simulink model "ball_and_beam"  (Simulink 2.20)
settings: Solver=FixedStepDiscrete  StartTime=0.0  StopTime=5.0  FixedStep=0.02  RelTol=1e-3  AbsTol=1e-6

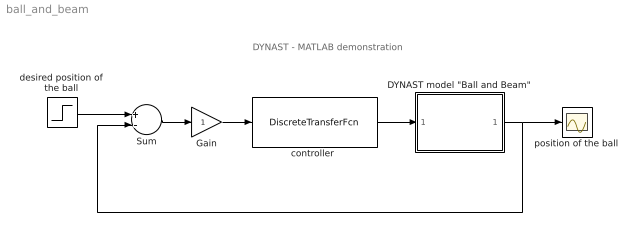
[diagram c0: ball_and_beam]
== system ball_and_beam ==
  note: DYNAST - MATLAB demonstration
  "DYNAST model \"Ball and Beam\"" : Subsystem
  Gain : Gain  Gain=1
  Sum : Sum  Inputs=+-
  "controller " : DiscreteTransferFcn  Numerator="[1010       -1020          10]"  Denominator="[1     1     0]"  SampleTime=0.02
  desired position of the ball : Step  Time=0  Before=0  After=0.25
  position of the ball : Scope
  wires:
  Sum/1 -> Gain/1
  Gain/1 -> "controller "/1
  "DYNAST model \"Ball and Beam\""/1(r) -> Sum/2, position of the ball/1
  "controller "/1 -> "DYNAST model \"Ball and Beam\""/1(theta)
  desired position of the ball/1 -> Sum/1

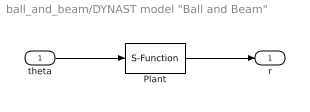
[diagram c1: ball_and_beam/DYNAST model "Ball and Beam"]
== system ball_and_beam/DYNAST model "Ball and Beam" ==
  theta : Inport  Port=1  PortWidth=-1  SampleTime=-1
  Plant : S-Function  FunctionName=dynPlantL  Parameters='%DYNAST%\examples\control\BallBeam.prb',0.02  PortCounts=[]  SFunctionModules=''
  r : Outport  Port=1
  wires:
  theta/1 -> Plant/1
  Plant/1 -> r/1
